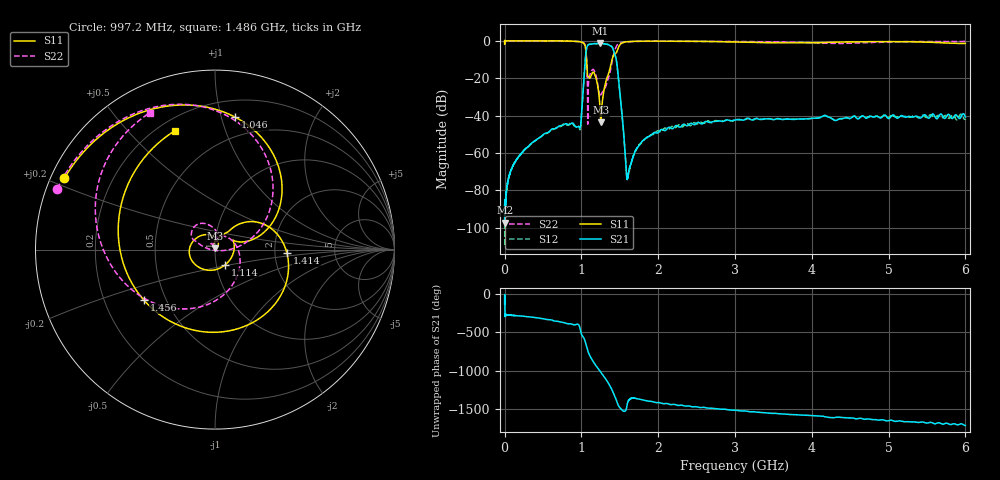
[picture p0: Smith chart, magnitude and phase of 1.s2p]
#  HZ  S  MA  R  50.00
! Rohde & Schwarz Vector Network Analyzer
! Rohde-Schwarz,ZNL6-2Port,1323001206101378,1.50.1.34-21.10.1.104
! Created: UTC 12/25/2023, 3:45:48 AM
! freq[Hz]  mag:S11  ang:S11  mag:S21  ang:S21  mag:S12  ang:S12  mag:S22  ang:S22
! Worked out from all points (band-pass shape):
!   6000 points, 5 kHz to 6 GHz, reference 50 ohm
!   highest |S21| = -1.39 dB at 1.24 GHz (marker M1); lowest = -97.3 dB at 1.005 MHz (marker M2)
!   |S21| within 3 dB of the highest: 1.066 GHz to 1.412 GHz (346.7 MHz wide, 28 % of centre)
!   lowest |S11| = -43.5 dB at 1.253 GHz (marker M3), VSWR 1.01, Z = 50 + j0.669 ohm
!   |S11| at or under -10 dB: 1.067 GHz to 1.398 GHz (331 MHz wide, 26.9 % of centre)
!   |S22| runs from -44.6 to 0.2 dB; largest |S21 - S12| = 0.044
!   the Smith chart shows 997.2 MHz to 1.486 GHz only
!   S11 on the Smith chart (normalised r, x): 997.2 MHz: 0.04, +0.22; 1.046 GHz: 0.33, +1.11; 1.114 GHz: 1.10, -0.19; 1.414 GHz: 2.33, -0.11; 1.456 GHz: 0.38, -0.28; 1.486 GHz: 0.26, +0.69
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5000  0.999 0.2  3.92e-05 -128.3  2.014e-05 17.9  1.002 -0.1
1005166  0.807 0.3  1.358e-05 -3.4  4.446e-05 67.0  0.9048 -0.6
6.801178e8  0.9977 -96.9  0.00472 8.1  0.004906 7.3  0.9951 -93.9
8.701493e8  0.9839 -140.8  0.006235 -29.1  0.006521 -33.8  0.9805 -139.4
9.971704e8  0.9282 154.7  0.008028 -151.9  0.007576 -149.6  0.9416 158.9
1.000171e9  0.9245 151.9  0.009811 -161.0  0.009511 -157.9  0.9387 156.5
1.046178e9  0.7463 81.3  0.2539 112.7  0.2407 104.0  0.787 92.4
1.11419e9  0.1021 -56.4  0.8059 -92.4  0.8164 -94.5  0.1313 155.4
1.171199e9  0.1302 158.6  0.8446 171.9  0.8356 170.8  0.152 109.2
1.240211e9  0.01839 44.5  0.8518 76.6  0.8532 74.8  0.03239 101.7
1.253213e9  0.006692 88.8  0.8505 58.8  0.8501 57.2  0.0355 120.2
1.300221e9  0.05631 82.0  0.8253 -5.5  0.8391 -7.0  0.05039 100.7
1.346228e9  0.1202 54.1  0.8054 -75.7  0.7934 -76.1  0.09468 49.0
1.41424e9  0.4015 -2.9  0.5872 152.8  0.586 152.2  0.3877 -121.7
1.456246e9  0.4861 -144.7  0.2983 50.8  0.2844 45.8  0.7202 157.4
1.486251e9  0.6991 108.6  0.08154 -24.0  0.086 -18.1  0.8446 115.5
1.607272e9  0.9531 -4.6  0.0002723 39.2  0.0002448 31.7  0.9452 30.4
2.000337e9  0.983 -70.1  0.003518 22.5  0.003945 18.2  0.9793 -51.3
3.000503e9  0.9369 -109.5  0.00765 -78.1  0.007775 -77.1  0.9625 -101.9
4.000668e9  0.8886 -115.6  0.008483 -147.9  0.008413 -147.9  0.8902 -118.6
5.000834e9  0.959 -122.8  0.008356 146.7  0.00881 148.9  0.9337 -124.2
6e9  0.8522 -124.2  0.009156 83.0  0.008069 98.2  0.97 -133.5
